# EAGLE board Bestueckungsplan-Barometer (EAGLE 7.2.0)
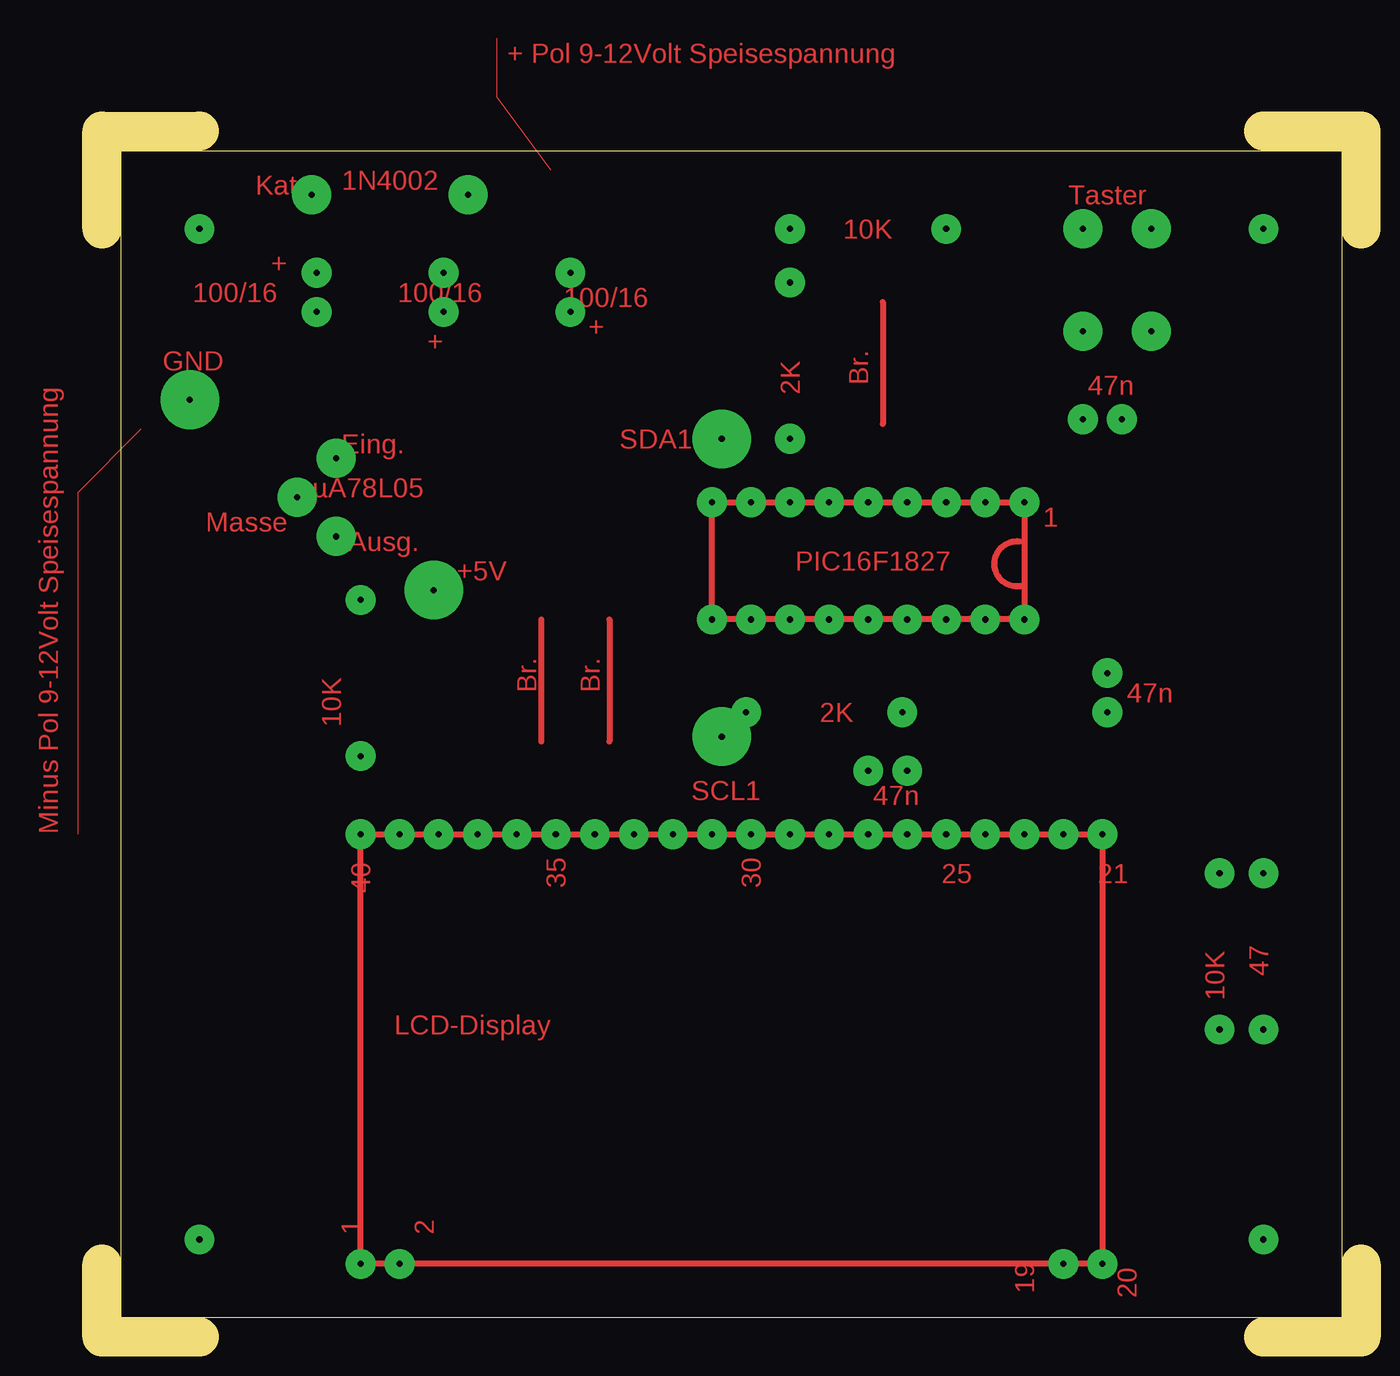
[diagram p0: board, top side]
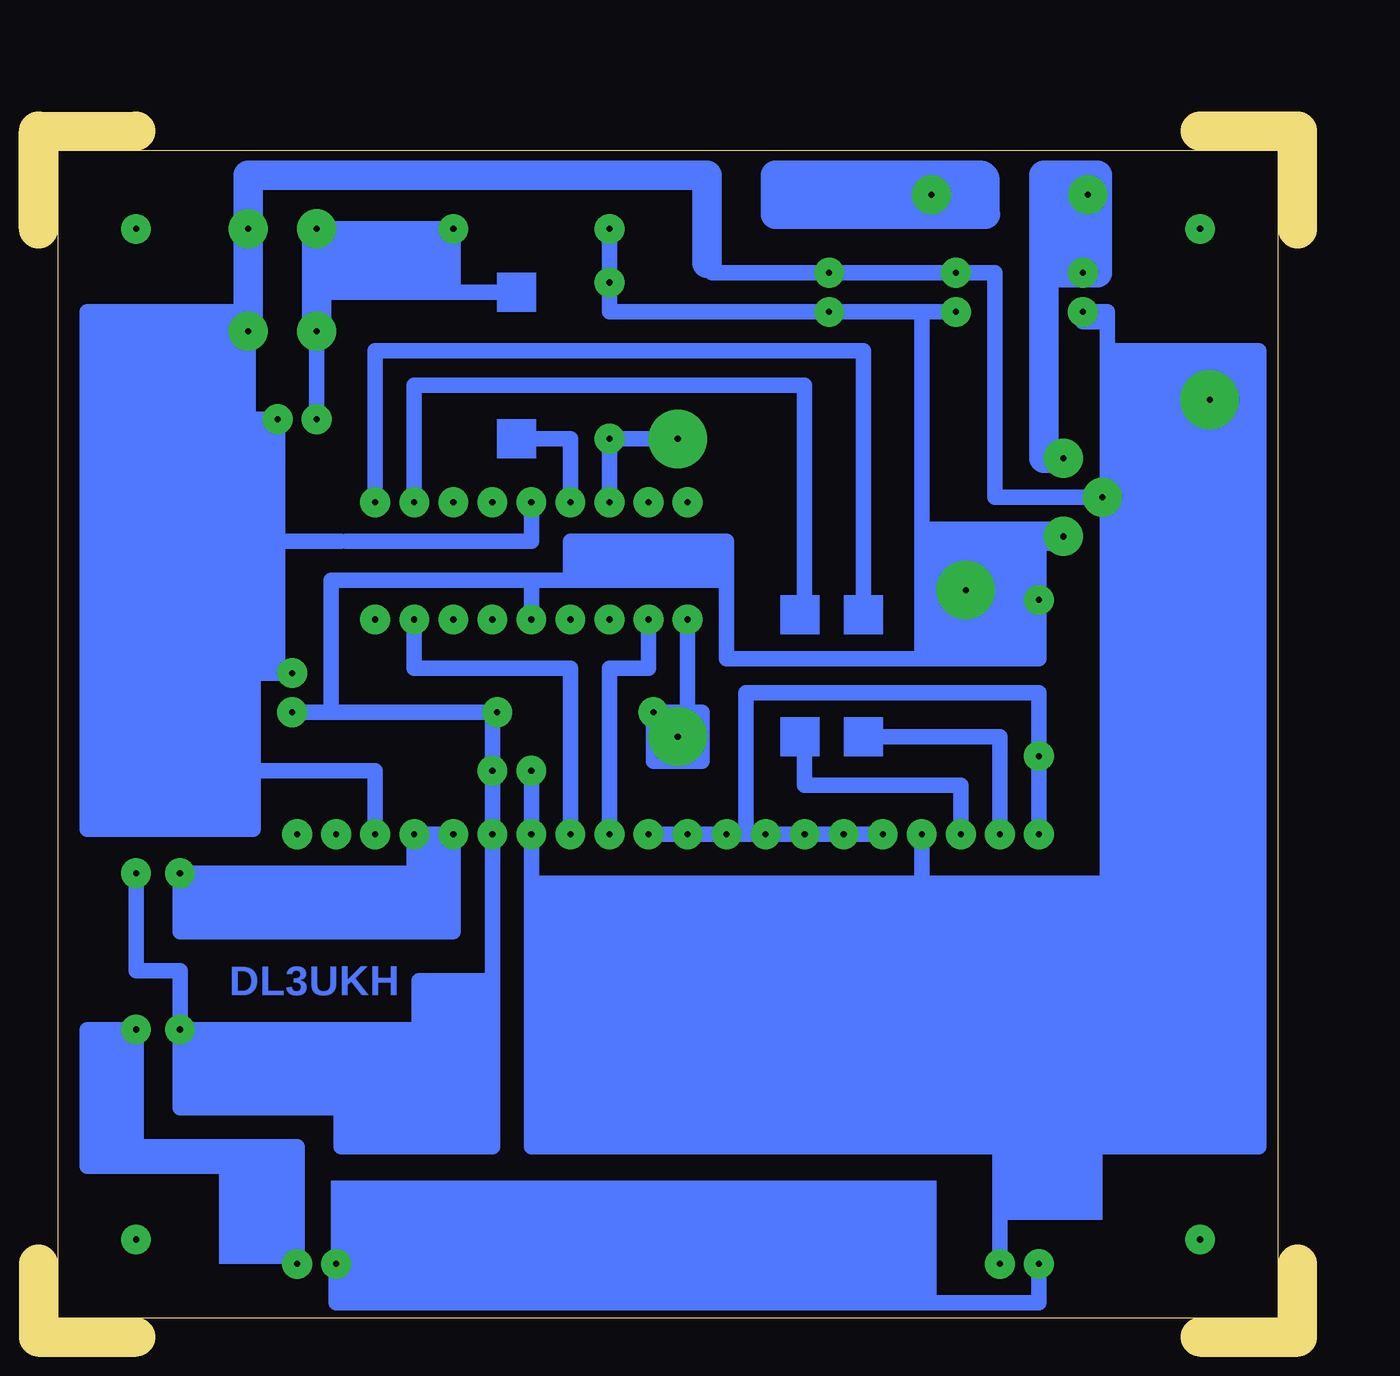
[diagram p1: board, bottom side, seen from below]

Size 81.91 x 78.42 mm. Coordinates in mm from the lower left corner, seen from the top.
Outline: 81.91,72.07 81.91,78.42 75.56,78.42
Outline: 81.91,4.76 81.91,0 75.56,0
Outline: 6.35,0 0,0 0,4.76
Outline: 0,72.07 0,78.42 6.35,78.42
Outline: 80.64,77.15 80.64,1.27 1.27,1.27 1.27,77.15 80.64,77.15
Copper layers (1*16): Top 0.035mm / dielectric 1.5mm / Bottom 0.035mm
Design rules "default": minimum track width 10mil, minimum drill 24mil, track to track 8mil, track to pad 8mil, pad to pad 8mil, via to via 8mil, smd to smd 8mil, copper to edge 40mil, drill to drill 8mil, minimum pad ring 10mil, minimum via ring 8mil, stop-mask expansion 4mil, vias tented up to drill 0mil, thermal gap 10mil

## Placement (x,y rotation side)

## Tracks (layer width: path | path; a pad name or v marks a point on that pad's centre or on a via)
S$2  (via drill 0.4 pad 1.93)
  other vias: 32.07,32.7
S$3  (via drill 0.4 pad 1.93)
  Bottom 1.016: v16.83,4.76 16.83,2.22 62.55,2.22 v62.55,4.76
S$4  (via drill 0.4 pad 1.93, 0.4 pad 2.54)
  Bottom 1.016: 11.75,54.61 v12.7,54.61 19.68,54.61 19.68,69.21 v22.22,69.21 38.1,69.21 | 11.75,54.61 11.75,27.3 13.33,14.92 | v19.37,4.76 19.37,14.92 | 19.37,14.92 49.85,14.92 | 49.85,14.92 49.85,24.45 | 49.85,28.89 49.85,29.53 | 49.85,29.53 v49.85,32.7 v49.85,36.83 | 49.85,14.92 49.85,12.38 13.65,12.38 | 13.33,14.92 19.37,14.92 | 13.33,14.92 13.33,12.38 2.54,12.38 2.54,64.14 12.38,64.14 | 41.59,28.89 40.64,28.89 40.64,24.45 49.85,24.45 | 41.59,28.89 49.85,28.89 | 49.85,28.89 49.85,24.45 | 41.59,27.62 41.59,28.89 | v5.71,60.96 12.38,64.14 | 11.75,54.61 12.38,64.14 | 12.06,29.53 49.85,29.53
S$5
  Bottom 1.016: 24.45,32.7 24.45,13.97
S$6  (via drill 0.4 pad 1.93, 0.4 pad 3.81)
  Bottom 1.016: v44.77,54.29 v44.77,58.42 v40.32,58.42
S$8  (via drill 0.4 pad 1.93)
  other vias: 6.35,6.35
S$9  (via drill 0.4 pad 1.93)
  other vias: 6.35,72.07
S$10
  Bottom 1.016: 65.41,75.25 65.41,75.88 | 65.41,75.88 68.58,75.88 | 51.12,75.56 48.26,75.88 | 48.26,75.88 65.41,75.88 | 48.26,75.88 38.42,75.88 38.42,75.56
  Bottom 1.93: 51.12,75.56 67.94,75.56 | 38.42,69.85 38.42,75.56 68.26,75.56 68.26,65.41
S$11  (via drill 0.4 pad 1.93)
  other vias: 34.61,32.7
S$12  (via drill 0.4 pad 1.93)
  other vias: 47.31,46.67
S$13
  Top 0.406: 28.57,46.67 28.57,38.74
S$14  (via drill 0.4 pad 1.93)
  Bottom 1.016: v44.77,32.7 44.77,43.5 42.23,43.5 v42.23,46.67
S$15  (via drill 0.4 pad 1.93)
  other vias: 24.45,32.7
S$16  (via drill 0.4 pad 1.93, 0.4 pad 2.54)
  Bottom 1.016: v63.82,72.07 v54.93,72.07 54.93,67.94 | 50.8,67.94 54.93,67.94 | 54.93,67.94 63.82,67.94 | v63.82,65.41 v63.82,59.69
  Bottom 1.93: v63.82,72.07 63.82,67.94 v63.82,65.41
S$17  (via drill 0.4 pad 1.93)
  Bottom 1.016: v49.85,54.29 49.85,51.75 61.91,51.75
S$18  (via drill 0.4 pad 1.93)
  other vias: 44.77,46.67
S$19  (via drill 0.4 pad 1.93, 0.4 pad 3.81, 0.5 pad 3.81)
  Bottom 1.016: v39.69,46.67 39.69,40.64 v41.91,40.64 | 38.74,40.64 v40.32,39.05 41.91,37.47 | 38.74,40.64 v41.91,40.64 | v41.91,40.64 41.91,37.47 | 38.74,40.64 38.74,37.47 41.91,37.47
  other vias: 42.23,54.29 -41.59,-5.71
S$20  (via drill 0.4 pad 1.93)
  other vias: 54.93,46.67
S$21
  Top 0.406: 33.02,46.67 33.02,38.74 | 50.8,67.31 50.8,59.37
S$22  (via drill 0.4 pad 1.93, 0.4 pad 2.54)
  Bottom 1.016: v68.26,65.41 68.26,59.69 v66.36,59.69 66.36,43.5
  Bottom 1.93: 71.12,65.41 v68.26,65.41 v68.26,72.07
S$23  (via drill 0.4 pad 3.81)
  other vias: 5.71,60.96
S$24  (via drill 0.4 pad 1.93)
  Bottom 1.016: v57.47,46.67 57.47,43.5 47.31,43.5 v47.31,32.7
S$25  (via drill 0.4 pad 1.93)
  other vias: 62.55,32.7
S$26  (via drill 0.4 pad 1.93)
  other vias: 65.09,32.7
S$27  (via drill 0.4 pad 3.81)
  other vias: 21.59,48.58
S$28  (via drill 0.4 pad 1.93)
  Bottom 1.016: v57.47,54.29 57.47,61.91 32.07,61.91 32.07,46.67
S$29  (via drill 0.4 pad 1.93)
  other vias: 75.56,6.35
S$30  (via drill 0.4 pad 1.93)
  Bottom 1.016: 60.01,26.35 72.71,26.35 v72.71,30.16 60.01,30.16 | 54.93,30.16 v54.93,32.7 v57.47,32.7 57.47,28.89 | 54.93,30.16 54.93,28.89 | 54.93,28.89 57.47,28.89 | 57.47,28.89 60.01,28.89 | 60.01,28.89 60.01,30.16 | 60.01,26.35 60.01,28.89 | 54.93,28.89 54.93,26.35 60.01,26.35 | 60.01,30.16 54.93,30.16
S$31
  Top 0: 29.21,75.88 25.72,80.64 25.72,84.45
S$32  (via drill 0.4 pad 1.93)
  Bottom 1.016: v47.31,54.29 47.31,58.42 50.8,58.42
S$33  (via drill 0.4 pad 1.93)
  Bottom 1.016: 28.26,46.67 28.26,64.14 60.01,64.14 v60.01,54.29
S$34  (via drill 0.4 pad 1.93)
  other vias: 75.56,72.07
S$35  (via drill 0.4 pad 1.93)
  Top 0.406: 60.01,48.9 60.01,54.29 v39.69,54.29 39.69,46.67 v60.01,46.67 60.01,48.9 | 60.01,48.9 arc-205 59.69,51.75
S$36
  Top 0: 2.54,59.05 -1.59,54.93 -1.59,32.7
S$37
  Bottom 1.016: 68.58,66.67 78.74,66.67 78.74,33.02 67.94,33.02 67.94,36.51
S$38  (via drill 0.4 pad 1.93)
  Bottom 1.016: v19.37,32.7 19.37,39.05 28.26,39.05
S$39  (via drill 0.4 pad 1.93)
  Bottom 1.016: v75.56,30.16 75.56,23.81 72.71,23.81 v72.71,20 | 57.15,19.37 57.15,23.18 52.39,23.18 | v72.71,20 52.71,20 | v72.71,20 72.71,14.92 52.39,14.92 | 52.39,23.18 v52.39,32.7 v52.39,36.83 52.39,40.64 | 62.23,15.24 62.23,12.38 52.39,12.38 52.39,14.92 | 52.39,23.18 52.39,14.92 | 49.53,49.21 62.87,49.21 62.87,40.64 | 52.39,40.64 60.64,40.64 62.87,40.64 | v52.07,40.64 52.39,40.64 | v65.41,40.64 62.87,40.64
S$40  (via drill 0.4 pad 1.93)
  other vias: 30.48,69.21
S$41  (via drill 0.4 pad 1.93)
  other vias: 52.39,54.29
S$42  (via drill 0.4 pad 1.93)
  Bottom 1.016: 66.67,54.29 67.94,54.29 | 67.94,54.29 77.47,54.29 | 77.47,54.29 78.74,54.29 | 77.47,54.29 77.47,36.83 | v60.01,32.7 60.01,36.83 67.94,36.83 | 67.94,36.83 78.42,36.83 | 67.94,54.29 67.94,36.83
S$43
  Bottom 1.016: 62.23,51.75 68.58,51.75
S$44  (via drill 0.4 pad 1.93)
  Bottom 1.016: 32.07,39.05 32.07,35.88 27.3,35.88 26.99,35.88 21.91,35.88 v21.91,32.7
S$45  (via drill 0.4 pad 1.93)
  other vias: 54.93,54.29
S$46  (via drill 0.4 pad 1.93)
  Bottom 1.016: v65.41,43.18 68.58,43.18
S$47  (via drill 0.4 pad 1.93)
  Top 0.406: v16.83,32.7 65.09,32.7 v65.09,4.76 16.83,4.76 v16.83,32.7
  Bottom 1.016: v16.83,32.7 v16.83,37.78 16.83,41.91 35.88,41.91 35.88,32.7 | 75.56,12.38 65.09,12.38 v65.09,4.76 | 75.56,12.38 v75.56,20 78.74,20 78.74,12.38 | 75.56,12.38 78.74,12.38 | 78.74,12.38 78.74,11.11 69.21,11.11 | v42.23,32.7 v37.15,32.7 35.88,32.7 | 35.88,32.7 v29.53,32.7 v26.99,32.7
S$48  (via drill 0.4 pad 1.93)
  other vias: 39.69,32.7
S$49  (via drill 0.4 pad 1.93, 0.4 pad 2.54)
  Bottom 1.93: 13.33,75.56 13.33,69.21 v13.97,69.21 14.92,69.21 | 14.92,75.56 14.92,73.34 | 14.92,73.34 v13.65,74.3 | 14.92,75.56 16.51,75.56 16.51,69.53 16.51,69.21 14.92,69.21 | 14.92,75.56 13.02,75.56 13.02,69.21 | 14.92,73.34 14.92,69.21 | 14.92,69.21 15.24,75.56
S$50
  Bottom 1.93: 20.32,73.02 33.97,73.02 33.97,75.56
S$51  (via drill 0.4 pad 1.93, 0.4 pad 2.54)
  Bottom 2.54: v23.81,74.3 20.95,75.25 24.13,75.25 | 24.13,75.25 v23.81,74.3 | v23.81,74.3 20.64,73.34 20.64,75.25 v23.81,74.3 | v23.81,74.3 29.84,73.34 33.66,75.25 24.13,75.25
  other vias: 5.71,60.96 5.71,60.96
S$52  (via drill 0.4 pad 1.93, 0.4 pad 2.54)
  Bottom 1.016: v16.83,47.94 16.83,44.13 22.22,44.13 | 22.22,44.13 37.15,44.13 37.15,49.21 | 37.15,49.21 47.31,49.21 | 47.31,49.21 49.85,49.21 v49.85,46.67 | v15.24,52.07 16.83,51.75 | 16.83,51.75 v16.83,47.94 | v16.83,47.94 22.22,47.94 | 22.22,47.94 22.22,44.13 | 16.83,51.75 22.22,51.75 | 22.22,51.75 22.22,47.94 | 22.22,51.75 24.45,44.45 24.45,66.67 | 37.15,49.21 37.15,51.75 47.31,51.75 47.31,49.21
  Bottom 1.93: 23.81,52.07 v15.24,52.07
S$53  (via drill 0.4 pad 2.54)
  Bottom 1.93: v15.24,57.15 16.51,57.15 16.51,68.9
S$54  (via drill 0.4 pad 1.93)
  Bottom 1.016: v22.22,66.67 v30.48,66.67 44.77,66.67 v44.77,68.58 v44.77,72.07
S$55
  Bottom 1.93: 11.75,63.5 11.75,62.87
S$56  (via drill 0.4 pad 1.93)
  Bottom 1.016: 12.38,28.26 12.38,64.45 12.38,66.04 | v13.97,66.67 12.38,66.67 12.38,66.04 | 13.97,66.04 12.38,66.04
S$57  (via drill 0.4 pad 1.93)
  other vias: 52.39,46.67
(copper drawn outside any net)
  shapes: Bottom area x36

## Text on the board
Top: + Pol 9-12Volt Speisespannung | 1N4002 | Kat | Taster | 10K | + | 100/16 | 100/16 | 100/16 | + | + | GND | 2K | Br. | 47n | SDA1 | Eing. | µA78L05 | 1 | Masse | Ausg. | +5V | PIC16F1827 | Br. | Br. | 2K | 47n | 10K | SCL1 | 47n | Minus Pol 9-12Volt Speisespannung | 40 | 35 | 30 | 25 | 21 | 47 | 10K | LCD-Display | 1 | 2 | 19 | 20
Bottom: DL3UKH
Pads: AUF BESTÜCKUNGS-SEITE GESEHEN
Dimension: 1 stck. Taster 1,0mm
tOrigins: 1N4148 | Katode | Anode | mit Kat | gekennzeichnet | hier im Plan | µA78L05 | PIC16F1827 | 1 | Links oben ist | immer PIN 1 | Ausg. | Eing. | Masse | BOHRUNGEN: | alles 0.8mm | 4Stck. Befestigungsbohr... 3,2mm | Leiterplatte: | 1,5mm dick | Cevausit | Runde / große Lötinseln sind | Viereckige Lötinseln sind | für die 4 Sensor- | für die 3 Brücken. | Anschlüsse des HP206c-Reichelt-Moduls. | Die 3 Brücken sind unterhalb | Hier auf der Leiterzug-Unterseite | auf der Leiterzug-Seite. | anlöten.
